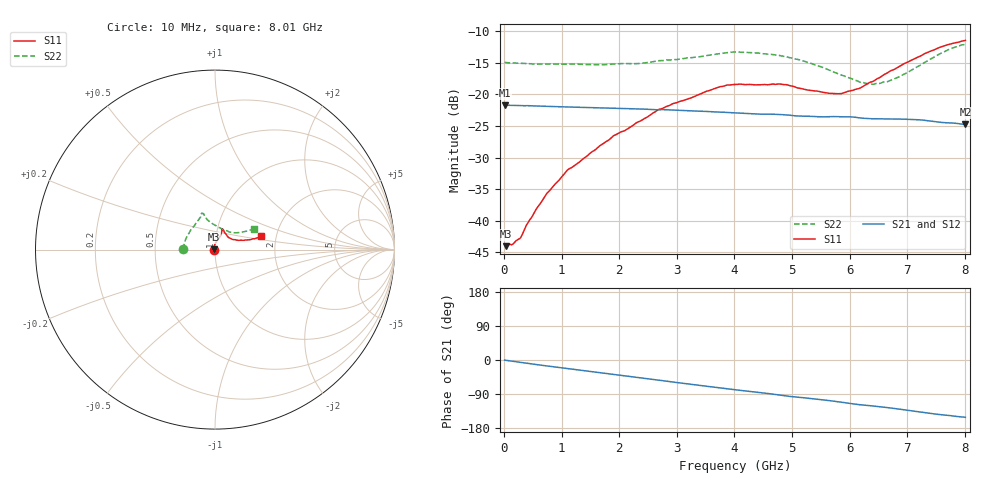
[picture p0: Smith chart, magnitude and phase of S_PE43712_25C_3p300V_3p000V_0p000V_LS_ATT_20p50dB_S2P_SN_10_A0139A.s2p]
! DEVICE ID: PE43712
! File Path: z:\PE43713\PE43713_CHAR_NOM_04292014\AMB\3p300\LS_ATT_20p50dB\PE43713_AMB_3p300V_3p000V_0p000V_LS_ATT_20p50dB_S2P_SN_10_A0139A.s2p
! Serial: 10
! Lot: A0139A
! Temp: 25C
! VDD: 3.300
! VSS: 0.000
! Control_Hi: 3.000
! Control_Lo: 0.000
! Attenuation Step: 20.50dB
! Port 1: RF1
! Port 2: RF2
! ThroughPath:1-2
! IDD: 0.0001467103
! ISS: -6.48e-008
#  Hz  S  RI  R  50
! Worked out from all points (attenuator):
!   801 points, 10 MHz to 8.01 GHz, reference 50 ohm
!   highest |S21| = -21.73 dB at 10 MHz (marker M1); lowest = -24.8 dB at 8.01 GHz (marker M2)
!   lowest |S11| = -44.0 dB at 30 MHz (marker M3), VSWR 1.01, Z = 49.4 + j0.137 ohm
!   |S11| at or under -10 dB: start of sweep to end of sweep
!   |S22| runs from -18.4 to -12.1 dB; largest |S21 - S12| = 0.0003
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1e7  -0.00654 0.00055  0.082 -0.000405  0.082 -0.000354  -0.1787 0.00118
3e7  -0.00614 0.00139  0.0819 -0.00101  0.082 -0.00103  -0.1781 0.00294
1.5e8  -0.00532 0.00376  0.0816 -0.00479  0.0816 -0.00478  -0.1766 0.011
2.7e8  -0.00462 0.00552  0.081 -0.00839  0.0811 -0.00844  -0.1749 0.0174
4.2e8  -0.00427 0.00875  0.0803 -0.0129  0.0802 -0.0129  -0.1729 0.0257
7.4e8  -0.00393 0.0159  0.0774 -0.0217  0.0774 -0.0217  -0.1678 0.0451
1.1e9  -0.00248 0.025  0.0731 -0.0307  0.0731 -0.0308  -0.1602 0.0653
1.35e9  -2.82e-05 0.0303  0.0698 -0.0365  0.0698 -0.0365  -0.154 0.0775
1.91e9  0.00875 0.0464  0.0608 -0.0482  0.0608 -0.0482  -0.135 0.1095
2.68e9  0.0269 0.0706  0.0453 -0.0604  0.0453 -0.0604  -0.1028 0.1528
3.72e9  0.0389 0.1068  0.0211 -0.0692  0.0211 -0.0692  -0.0764 0.1942
4.01e9  0.0403 0.1127  0.0143 -0.0699  0.0143 -0.0699  -0.0751 0.2022
4.79e9  0.044 0.1124  -0.00308 -0.0691  -0.00306 -0.0691  -0.061 0.1929
5.35e9  0.0564 0.0908  -0.0142 -0.0653  -0.0142 -0.0653  -0.0451 0.1684
5.87e9  0.0771 0.0664  -0.0244 -0.0618  -0.0243 -0.0618  -0.00832 0.1411
6.17e9  0.0954 0.0577  -0.0304 -0.0575  -0.0303 -0.0575  0.0208 0.1235
6.32e9  0.1087 0.0553  -0.0323 -0.0557  -0.0322 -0.0556  0.0386 0.1152
6.68e9  0.1413 0.0518  -0.0376 -0.0515  -0.0375 -0.0514  0.0807 0.0985
7e9  0.1706 0.0533  -0.0429 -0.0467  -0.0428 -0.0467  0.1145 0.0936
7.54e9  0.2243 0.0618  -0.0485 -0.0358  -0.0484 -0.0358  0.1777 0.1034
7.81e9  0.2442 0.0698  -0.0502 -0.0314  -0.0501 -0.0314  0.2055 0.1127
8.01e9  0.2554 0.0761  -0.0505 -0.0278  -0.0505 -0.0279  0.2185 0.1163
